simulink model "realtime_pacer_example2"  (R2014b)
settings: Solver=ode3  StartTime=0.0  StopTime=60  FixedStep=0.05  RelTol=1e-3
model workspace (MAT data in the model file):
  Var = 0
libraries: realtime_pacer_lib x2

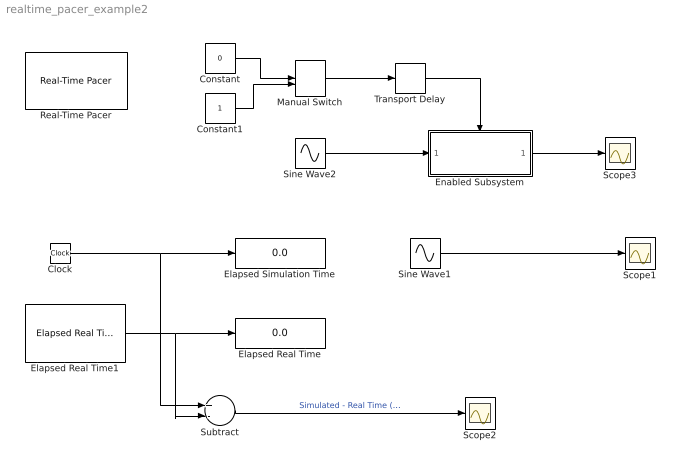
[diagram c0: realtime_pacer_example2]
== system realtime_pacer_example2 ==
  Clock : Clock
  Constant : Constant  Value=0
  Constant1 : Constant
  Elapsed Real Time : Display
  Elapsed Real Time1 : realtime_pacer_lib/Elapsed Real Time
  Elapsed Simulation Time : Display
  Enabled Subsystem : Subsystem  TreatAsAtomicUnit=on
  Manual Switch : ManualSwitch
  Real-Time Pacer : realtime_pacer_lib/Real-Time Pacer  simTimePerRealTime=1
  Scope1 : Scope
  Scope2 : Scope
  Scope3 : Scope
  Sine Wave1 : Sin  Frequency=2*pi*0.5  SampleTime=0
  Sine Wave2 : Sin  Frequency=2*pi*0.5  SampleTime=0
  Subtract : Sum  Inputs=+-
  Transport Delay : TransportDelay  DelayTime=5
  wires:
  Clock/1 -> Elapsed Simulation Time/1, Subtract/1
  Subtract/1 -> Scope2/1  "Simulated - Real Time (seconds)"
  Elapsed Real Time1/1 -> Elapsed Real Time/1, Subtract/2
  Sine Wave1/1 -> Scope1/1
  Constant/1 -> Manual Switch/1
  Transport Delay/1 -> Enabled Subsystem/Enable
  Sine Wave2/1 -> Enabled Subsystem/1(In1)
  Enabled Subsystem/1(Out1) -> Scope3/1
  Manual Switch/1 -> Transport Delay/1
  Constant1/1 -> Manual Switch/2

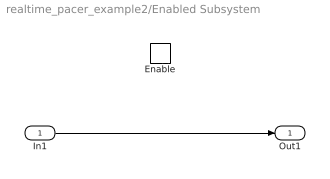
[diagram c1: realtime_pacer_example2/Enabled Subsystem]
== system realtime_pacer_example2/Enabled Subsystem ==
  In1 : Inport
  Enable : EnablePort
  Out1 : Outport
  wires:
  In1/1 -> Out1/1
